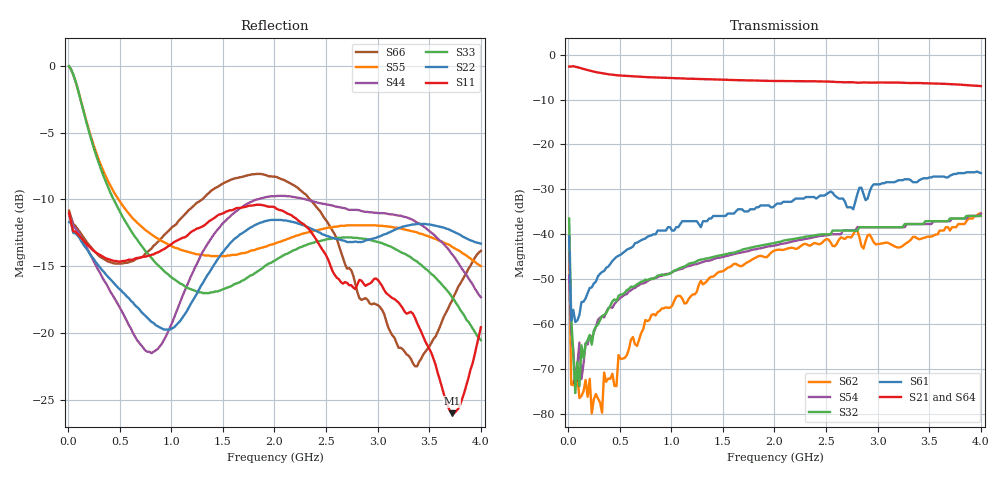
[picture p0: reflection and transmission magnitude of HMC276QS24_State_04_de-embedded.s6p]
! Hittite Microwave Corporation
! 20 Alpha Road
! Chelmsford, MA 01824
! Tel: 978-250-3343
! Fax: 978-250-3373
! Device: HMC276QS24, 0.7-3.0 GHz, GaAS MMIC 4x2 Switch Matrix in 24-lead QSOP package
! Misc: Data was de-embedded to package pins.
!  Port 1 = OP1
!  Port 2 = VL
!  Port 3 = VH
!  Port 4 = HH
!  Port 5 = HL
!  Port 6 = OP2
!  Vdd = +5 V
!  Vctl = 0 V[Logic 0] / +5 V[Logic 1]
!  State 04,  VL to OP1,  HH to OP2
!  Control Lines (Logic)
!  HV 1 = 0, Tone 1 = 0
!  HV 2 = 1, Tone 2 = 1
!  Data reformated to new Touchstone file format - Wed Jan 10 14:32:42 2007
# MHz S DB R 50
! 6 Port Network Data
! freq  dbS11  angS11  dbS12  angS12  dbS13  angS13  dbS14  angS14
!  dbS15  angS15  dbS16  angS16
!  dbS21  angS21  dbS22  angS22
!  dbS23  angS23  dbS24  angS24  dbS25  angS25  dbS26  angS26
!  dbS31  angS31  dbS32  angS32  dbS33  angS33  dbS34  angS34
!  dbS35  angS35  dbS36  angS36
!  dbS41  angS41  dbS42  angS42
!  dbS43  angS43  dbS44  angS44  dbS45  angS45  dbS46  angS46
!  dbS51  angS51  dbS52  angS52  dbS53  angS53  dbS54  angS54
!  dbS55  angS55  dbS56  angS56
!  dbS61  angS61  dbS62  angS62
!  dbS63  angS63  dbS64  angS64  dbS65  angS65  dbS66  angS66
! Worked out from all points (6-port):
!   201 points, 10 MHz to 4 GHz, reference 50 ohm
!   strongest paths, dB at 10 MHz, 1.008 GHz, 2.005 GHz, 3.002 GHz, 4 GHz:
!     S21: -2.7, -5.2, -5.8, -6.2, -7.0
!     S64: -2.6, -5.4, -6.2, -6.3, -7.0
!     S61: -40.5, -39.2, -33.6, -28.9, -26.4
!     S32: -36.5, -48.4, -41.9, -38.4, -35.9
!     S54: -49.2, -48.5, -42.5, -38.4, -35.4
!     S62: -43.4, -56.0, -43.6, -42.2, -35.4
!   lowest |S11| = -26.0 dB at 3.721 GHz (marker M1), VSWR 1.11, Z = 48.7 + j4.78 ohm
!   |S11| at or under -10 dB: start of sweep to end of sweep
